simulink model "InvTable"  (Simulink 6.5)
settings: Solver=FixedStepDiscrete  StartTime=0.0  StopTime=inf  FixedStep=samplePeriod  RelTol=1e-3
PreLoadFcn:
  | initialize
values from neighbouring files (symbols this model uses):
  accelCanon = 9810    [initialize.m]
  aInv = bFwd / bFwd(1)    [initialize.m]
  bInv = aFwd / bFwd(1)    [initialize.m]
  flowCanon = 1.666667e+04    (= 16666.67)    [initialize.m]    (also in Copy of initialize.m)
  forceCanon = 1    [initialize.m]    (also in Copy of initialize.m)
  friction = 5			 				* 0.155000	 				* 0.00444822 				* area1    (= 2.71252900422)    [initialize.m]
  gasConstant = 1.8    [initialize.m]    (also in Copy of initialize.m)
  iactParams = [actParams, dfGain, solver]    [initialize.m]
  lengthCanon = 1    [initialize.m]    (also in Copy of initialize.m)
  massCanon = 1e-06    [initialize.m]    (also in Copy of initialize.m)
  maxOilVolume = volume * (1 - (precharge/supplyPress)^(1/gasConstant))    (= 211.391477114)    [initialize.m]    (also in Copy of initialize.m)
  precharge = 3000		 				* 6.894757e-03    (= 20.684271)    [initialize.m]    (also in Copy of initialize.m)
  pumpFlow = 1e20    (= 1e+20)    [initialize.m]    (also in Copy of initialize.m)
  returnPress = 3			 				* 0.1    (= 0.3)    [initialize.m]    (also in Copy of initialize.m)
  rigidMass = 32900		 				+ (   3596	 				   +   528	 				   +    43	 				   +   122)	 				* 0.453592    (= 34845.456088)    [initialize.m]
  supplyPress = 280		 				* 0.1    (= 28)    [initialize.m]    (also in Copy of initialize.m)
  velocCanon = 1    [initialize.m]    (also in Copy of initialize.m)
  volume = 15.15		 				+ (  45		 				    * 2		 				   + 30		 				    * 6 )	 				* 5    (= 1365.15)    [initialize.m]    (also in quake.m = volume / 231.0; Copy of initialize.m)
  volumeCanon = 1e+06    (= 1000000)    [initialize.m]    (also in Copy of initialize.m)
  yieldDispl = 1.0    (= 1)    [initialize.m]
undefined symbols (not defined in the file or in its folder): DiscIntNeverNeededParam

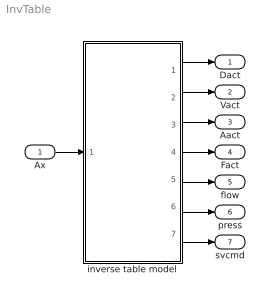
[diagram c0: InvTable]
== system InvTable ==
  Ax : Inport  PortDimensions=1
  inverse table model : Subsystem
  Dact : Outport
  Vact : Outport  Port=2
  Aact : Outport  Port=3
  Fact : Outport  Port=4
  flow : Outport  Port=5
  press : Outport  Port=6
  svcmd : Outport  Port=7
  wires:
  Ax/1 -> inverse table model/1(Ax)
  inverse table model/1(Dact) -> Dact/1
  inverse table model/2(Vact) -> Vact/1
  inverse table model/3(Aact) -> Aact/1
  inverse table model/4(Fact) -> Fact/1
  inverse table model/5(flow) -> flow/1
  inverse table model/6(press) -> press/1
  inverse table model/7(svcmd) -> svcmd/1

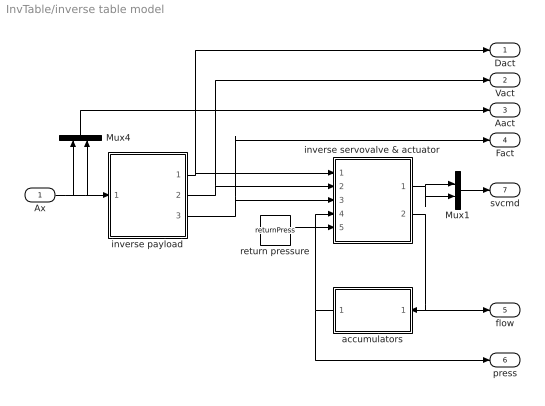
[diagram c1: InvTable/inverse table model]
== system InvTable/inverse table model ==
  Ax : Inport
  Mux1 : Mux  Inputs=2
  Mux4 : Mux  Orientation=up  Inputs=2
  accumulators : Subsystem  Orientation=left
  inverse payload : Subsystem
  inverse servovalve & actuator : Subsystem  mask(Inverse actuator){params=iactParams}
      mask prompts: params "Parameter vector"
  return pressure : Constant  Value=returnPress  OutDataType=sfix(16)  ConRadixGroup=Use specified scaling  OutScaling=2^0  SampleTime=inf  FramePeriod=inf
  Dact : Outport
  Vact : Outport  Port=2
  Aact : Outport  Port=3
  Fact : Outport  Port=4
  flow : Outport  Port=5
  press : Outport  Port=6
  svcmd : Outport  Port=7
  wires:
  Ax/1 -> Mux4/1, inverse payload/1(accel), Mux4/2
  Mux4/1 -> Aact/1
  accumulators/1(press) -> press/1, inverse servovalve & actuator/4(spl press)
  return pressure/1 -> inverse servovalve & actuator/5(rtn press)
  inverse servovalve & actuator/2(flow) -> accumulators/1(flow), flow/1
  inverse servovalve & actuator/1(cmd) -> Mux1/1, Mux1/2
  Mux1/1 -> svcmd/1
  inverse payload/1(displ) -> Dact/1, inverse servovalve & actuator/1(displ)
  inverse payload/2(veloc) -> Vact/1, inverse servovalve & actuator/2(veloc)
  inverse payload/3(force) -> Fact/1, inverse servovalve & actuator/3(force)

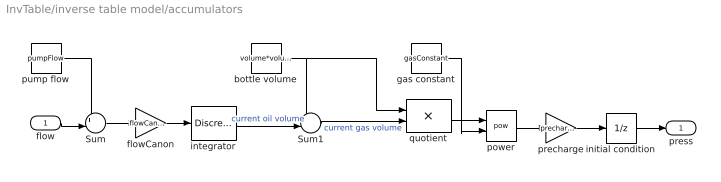
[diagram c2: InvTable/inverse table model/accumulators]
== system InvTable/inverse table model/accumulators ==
  flow : Inport
  Sum : Sum  Inputs=+-|
  Sum1 : Sum  Inputs=+-|
  bottle volume : Constant  Value=volume*volumeCanon  OutDataType=sfix(16)  ConRadixGroup=Use specified scaling  OutScaling=2^0  SampleTime=inf  FramePeriod=inf
  flowCanon : Gain  Gain=flowCanon
  gas constant : Constant  Value=gasConstant  OutDataType=sfix(16)  ConRadixGroup=Use specified scaling  OutScaling=2^0  SampleTime=inf  FramePeriod=inf
  initial condition : UnitDelay  X0=supplyPress  SampleTime=-1
  integrator : DiscreteIntegrator  InitialCondition=maxOilVolume*volumeCanon  SampleTime=-1  LimitOutput=on  UpperSaturationLimit=maxOilVolume*volumeCanon  LowerSaturationLimit=0  ICPrevOutput=DiscIntNeverNeededParam  ICPrevScaledInput=DiscIntNeverNeededParam
  power : Math  Operator=pow
  precharge : Gain  Gain=precharge
  pump flow : Constant  Value=pumpFlow  OutDataType=sfix(16)  ConRadixGroup=Use specified scaling  OutScaling=2^0  SampleTime=inf  FramePeriod=inf
  quotient : Product  Inputs=*/
  press : Outport
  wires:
  pump flow/1 -> Sum/1
  Sum/1 -> flowCanon/1
  bottle volume/1 -> Sum1/1, quotient/1
  gas constant/1 -> power/2
  power/1 -> precharge/1
  precharge/1 -> initial condition/1
  Sum1/1 -> quotient/2  "current gas volume"
  quotient/1 -> power/1
  integrator/1 -> Sum1/2  "current oil volume"
  flow/1 -> Sum/2
  flowCanon/1 -> integrator/1
  initial condition/1 -> press/1

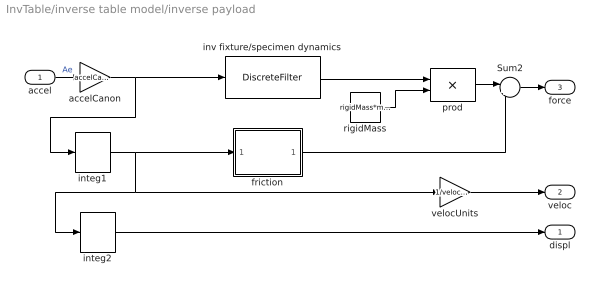
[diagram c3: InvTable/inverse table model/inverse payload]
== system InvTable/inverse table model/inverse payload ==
  accel : Inport
  Sum2 : Sum  Inputs=|++
  accelCanon : Gain  Gain=accelCanon
  friction : Subsystem  mask{friction=friction*forceCanon, yieldDispl=yieldDispl*lengthCanon, hysteresis=0}
      mask prompts: friction "Sliding friction"; yieldDispl "Equiv. yield displacement (in)"; hysteresis "Hysteresis constant"
  integ1 : DiscreteIntegrator  IntegratorMethod=Integration: Backward Euler  SampleTime=-1  ICPrevOutput=DiscIntNeverNeededParam  ICPrevScaledInput=DiscIntNeverNeededParam
  integ2 : DiscreteIntegrator  IntegratorMethod=Integration: Backward Euler  SampleTime=-1  ICPrevOutput=DiscIntNeverNeededParam  ICPrevScaledInput=DiscIntNeverNeededParam
  inv fixture/specimen dynamics : DiscreteFilter  Numerator=bInv  Denominator=aInv  SampleTime=-1
  prod : Product  Inputs=**
  rigidMass : Constant  Value=rigidMass*massCanon  OutDataType=sfix(16)  ConRadixGroup=Use specified scaling  OutScaling=2^0  SampleTime=inf  FramePeriod=inf
  velocUnits : Gain  Gain=1/velocCanon
  displ : Outport
  veloc : Outport  Port=2
  force : Outport  Port=3
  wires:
  rigidMass/1 -> prod/2
  prod/1 -> Sum2/1
  inv fixture/specimen dynamics/1 -> prod/1
  friction/1(force) -> Sum2/2
  integ2/1 -> displ/1
  integ1/1 -> friction/1(veloc), integ2/1, velocUnits/1
  accelCanon/1 -> integ1/1, inv fixture/specimen dynamics/1
  accel/1 -> accelCanon/1  "Ae"
  Sum2/1 -> force/1
  velocUnits/1 -> veloc/1

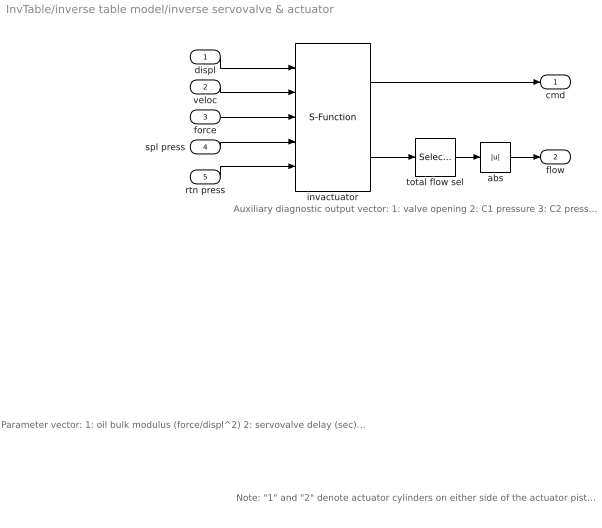
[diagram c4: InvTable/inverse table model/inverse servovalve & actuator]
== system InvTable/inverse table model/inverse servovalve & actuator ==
  note: Parameter vector: 1: oil bulk modulus (force/displ^2) 2: servovalve delay (sec) 3: servovalve overlap 4: rated pressure (force/displ^2) 5: rated flow at rated pressure (displ^3/sec) 6: nominal flow at rated pressure (displ^3/sec) 7: actuator piston area 1 (displ^2) 8: actuator piston area 2 (displ^2) 9: actuator usable stroke 1 (displ) 10: actuator usable stroke 2 (displ) 11: actuator end cushion length 1 (displ) 12: actuator end cushion length 2 (displ) 13: additional port volume 1 (displ^3) 14: additional port volume 1 (displ^3) 15: actuator parasitic damping factor 16: cross-chamber leakage factor (flow/press) 17: ratio port openings according to area 18: sample period (sec) Conversion factors used for converting signals from external (user) to internal (canonical) units: 19: displacement 20: velocity 21: force 22: pressure 23: flow Other: 24: delta-F feedback gain 25: inverse solver (0: exact, 1: approx)
  note: Note: "1" and "2" denote actuator cylinders on either side of the actuator piston. With positive valve drive, oil is ported into cylinder 1, resulting in positive displacement.
  note: Auxiliary diagnostic output vector: 1: valve opening 2: C1 pressure 3: C2 pressure 4: delta pressure 5: force 6: velocity 7: C1 flow 8: C2 flow 9: total flow 10: kinematic flow 11: compressibility flow 12: leakage flow 13: C1 oilspring displacement 14: C2 oilspring displacement 15: C1 oilspring velocity 16: C2 oilspring velocity 17: iteration error
  displ : Inport
  veloc : Inport  Port=2
  force : Inport  Port=3
  spl press : Inport  Port=4
  rtn press : Inport  Port=5
  abs : Abs  SaturateOnIntegerOverflow=on  SampleTime=-1
  invactuator : S-Function  FunctionName=InvActuator  Parameters=params
  total flow sel : Selector  InputType=Vector  ElementSrc=Internal  Elements=9  RowSrc=Internal  Rows=1  ColumnSrc=Internal  Columns=1  IndexIsStartValue=off
  cmd : Outport
  flow : Outport  Port=2
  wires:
  spl press/1 -> invactuator/4
  rtn press/1 -> invactuator/5
  displ/1 -> invactuator/1
  invactuator/1 -> cmd/1
  veloc/1 -> invactuator/2
  force/1 -> invactuator/3
  invactuator/2 -> total flow sel/1
  total flow sel/1 -> abs/1
  abs/1 -> flow/1

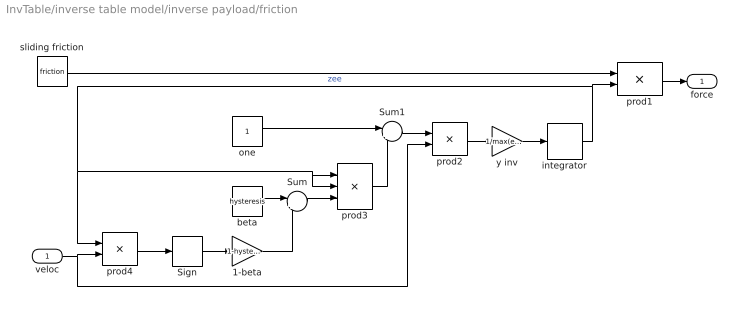
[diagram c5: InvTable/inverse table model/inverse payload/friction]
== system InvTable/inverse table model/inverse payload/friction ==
  veloc : Inport
  1-beta : Gain  Gain=1-hysteresis
  Sign : Signum
  Sum : Sum  Inputs=|++
  Sum1 : Sum  Inputs=|+-
  beta : Constant  Value=hysteresis  OutDataType=sfix(16)  ConRadixGroup=Use specified scaling  OutScaling=2^0  SampleTime=inf  FramePeriod=inf
  integrator : DiscreteIntegrator  SampleTime=-1  LimitOutput=on  UpperSaturationLimit=1  LowerSaturationLimit=-1  ICPrevOutput=DiscIntNeverNeededParam  ICPrevScaledInput=DiscIntNeverNeededParam
  one : Constant  Value=1  OutDataType=sfix(16)  ConRadixGroup=Use specified scaling  OutScaling=2^0  SampleTime=inf  FramePeriod=inf
  prod1 : Product
  prod2 : Product
  prod3 : Product  Inputs=3
  prod4 : Product
  sliding friction : Constant  Value=friction  OutDataType=sfix(16)  ConRadixGroup=Use specified scaling  OutScaling=2^0  SampleTime=inf  FramePeriod=inf
  y inv : Gain  Gain=1/max(eps, yieldDispl)
  force : Outport
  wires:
  integrator/1 -> prod3/2, prod3/1, prod4/1, prod1/2  "zee"
  y inv/1 -> integrator/1
  prod2/1 -> y inv/1
  Sum1/1 -> prod2/1
  prod3/1 -> Sum1/2
  one/1 -> Sum1/1
  Sum/1 -> prod3/3
  beta/1 -> Sum/1
  1-beta/1 -> Sum/2
  Sign/1 -> 1-beta/1
  prod4/1 -> Sign/1
  veloc/1 -> prod2/2, prod4/2
  prod1/1 -> force/1
  sliding friction/1 -> prod1/1
